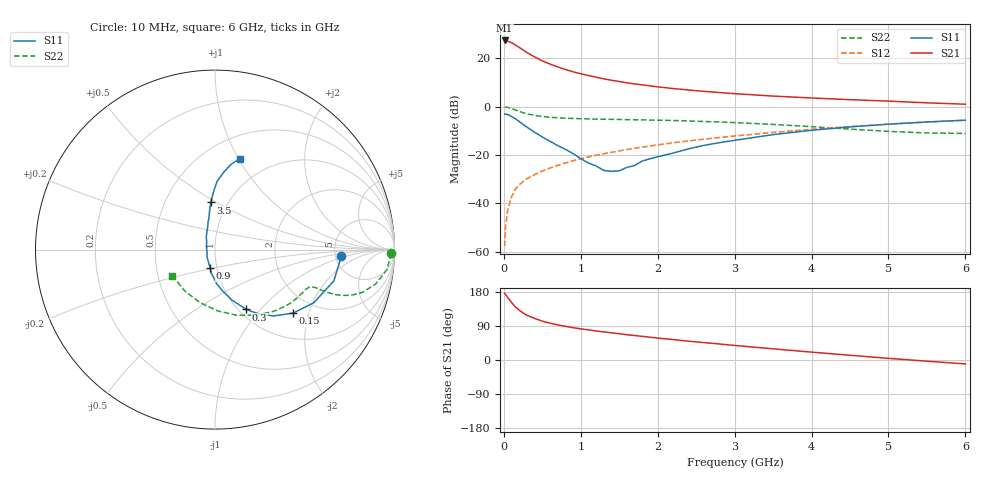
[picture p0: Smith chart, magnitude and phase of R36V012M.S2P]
! SIEMENS Small Signal Semiconductors
! BFR181
! Si NPN RF Bipolar Junction Transistor in SOT23
! VCE = 6 V  IC = 12 mA
! Common Emitter S-Parameters:  May  1996
# GHz  S  MA  R  50
!  f  S11  S21  S12  S22
! GHz  MAG  ANG  MAG  ANG  MAG  ANG  MAG  ANG
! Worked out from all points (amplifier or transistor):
!   36 points, 10 MHz to 6 GHz, reference 50 ohm
!   highest |S21| = 27.4 dB at 10 MHz (marker M1)
!   |S21| within 3 dB of that: start of sweep to 205.5 MHz
!   unconditionally stable (mu >= 1): 773.3 MHz to 2.675 GHz
!   at 250 MHz: K = 0.64, MSG = 27.2 dB, |S12| = -31.0 dB
!   at 1.4 GHz: K = 1.05, MAG = 13.5 dB, |S12| = -18.9 dB
!   at 6 GHz: K = 0.86, MSG = 3.3 dB, |S12| = -5.6 dB
!   S11 on the Smith chart (normalised r, x): 10 MHz: 5.55, -0.83; 150 MHz: 1.54, -1.59; 300 MHz: 1.08, -0.84; 900 MHz: 0.93, -0.19; 3.5 GHz: 0.83, +0.47; 6 GHz: 0.72, +1.01
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0.01  0.7006 -3.1  23.37 176.1  0.0013 95.9  0.9818 -1.2
0.02  0.6975 -5.7  23.01 173.3  0.0031 87.3  0.9771 -2.7
0.05  0.6848 -14.7  22.58 165.2  0.0072 84.0  0.9643 -6.7
0.1  0.6255 -28.2  21.03 152.0  0.0137 77.3  0.9139 -12.2
0.15  0.561 -39.1  18.8 140.2  0.0196 73.0  0.8538 -16.3
0.2  0.4924 -48.7  16.77 131.4  0.0242 71.1  0.7986 -18.6
0.25  0.4288 -56.2  14.82 123.9  0.0281 69.5  0.7491 -19.9
0.3  0.3759 -62.5  13.16 118.1  0.0323 69.7  0.7118 -20.6
0.4  0.296 -71.5  10.68 109.7  0.0393 69.9  0.6593 -20.9
0.5  0.2353 -79.4  8.846 102.5  0.0464 69.8  0.6254 -20.8
0.6  0.1919 -86.9  7.596 97.2  0.0538 70.6  0.6027 -20.7
0.7  0.1568 -92.5  6.629 92.8  0.0611 71.2  0.5874 -20.9
0.9  0.1065 -104.3  5.256 85.3  0.0761 71.1  0.5695 -21.5
1.1  0.0681 -126.7  4.397 79.5  0.0909 70.9  0.5573 -22.8
1.3  0.0477 -156.8  3.757 74.1  0.1064 70.5  0.5488 -24.4
1.6  0.0554 150.1  3.109 66.7  0.1294 69.1  0.5391 -27.5
2.2  0.1095 114.4  2.365 53.9  0.1785 65.6  0.5159 -35.2
2.8  0.1795 100.8  1.959 42.3  0.2297 61.0  0.4823 -44.4
3.5  0.2635 95.2  1.653 29.5  0.2925 54.6  0.4286 -58.4
4.5  0.381 88.2  1.393 12.5  0.3879 43.8  0.3423 -87.3
5.5  0.4818 79.5  1.199 -3.1  0.48 31.2  0.2855 -126.2
6  0.5248 74.9  1.122 -10.3  0.5229 24.3  0.2787 -148.3
